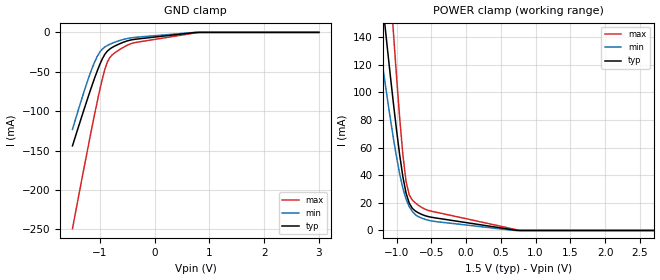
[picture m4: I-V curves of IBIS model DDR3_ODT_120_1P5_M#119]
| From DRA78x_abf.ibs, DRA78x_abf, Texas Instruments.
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| Model based on original model for DDR_SEIOPB_V
|   Sub model DDR3_ODT_120_1P5
[model]   DDR3_ODT_120_1P5_M#119
|[Description]  [1.5V-INPUT-X-X]
|   , ,
|[Input Load]
|[Output Drive]
|Voltage   1.5V
|Mode   INPUT
Model_type   Input
Polarity   Non-Inverting
Vinl = 0.65
Vinh = 0.85
C_comp   1p   0.5p   1.75p
[Receiver Thresholds]
Tslew_ac = 0.5n
Vth = 0.75
Vth_max = 0.7875
Vth_min = 0.675
Vinh_ac = 0.175
Vinh_dc = 0.1
Vinl_ac = -0.175
Vinl_dc = -0.1
[Temperature Range]   25   125   -40
[Voltage Range]   1.5   1.425   1.575
[POWER_clamp]
-1.5V     313.5mA    230.7mA    499.5mA
-1.273V   199.8mA    145.4mA    317.8mA
-1.182V   155.6mA    112.6mA    246.7mA
-1.136V   133.9mA    96.79mA    211.7mA
-1.045V   92.18mA    66.78mA    143.6mA
-954.5mV  54.51mA    40.82mA    81.12mA
-909.1mV  38.89mA    30.54mA    54.77mA
-863.6mV  27.13mA    22.75mA    35.57mA
-818.2mV  19.83mA    17.32mA    25.73mA
-727.3mV  14.01mA    11.35mA    19.86mA
772.7mV   0A         0A         0A
3V        0A         0A         0A
[GND_clamp]
-1.5V     -144mA     -123.1mA   -249.1mA
-1.318V   -104.1mA   -81.62mA   -182.5mA
-1.182V   -75.27mA   -53.07mA   -133.7mA
-1.091V   -57.04mA   -36.82mA   -102.3mA
-1V       -40.52mA   -24.95mA   -72.54mA
-909.1mV  -27.83mA   -18.53mA   -46.98mA
-863.6mV  -23.8mA    -16.61mA   -37.72mA
-772.7mV  -19.02mA   -13.67mA   -28.41mA
-590.9mV  -13.06mA   -9.333mA   -19.82mA
-409.1mV  -9.294mA   -6.738mA   -13.81mA
772.7mV   0A         0A         -328.7uA
3V        0A         0A         0A
